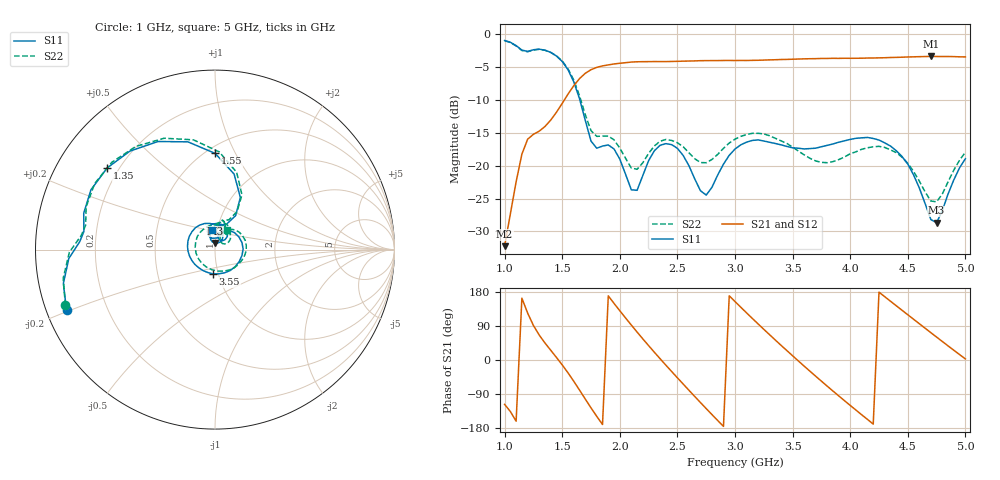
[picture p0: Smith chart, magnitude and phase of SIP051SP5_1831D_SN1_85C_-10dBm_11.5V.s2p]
# GHz  S  dB  R  50
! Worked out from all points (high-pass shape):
!   81 points, 1 GHz to 5 GHz, reference 50 ohm
!   highest |S21| = -3.41 dB at 4.7 GHz (marker M1); lowest = -32.2 dB at 1 GHz (marker M2)
!   |S21| within 3 dB of the highest: 1.673 GHz to end of sweep
!   lowest |S11| = -28.7 dB at 4.75 GHz (marker M3), VSWR 1.08, Z = 49.7 + j3.66 ohm
!   |S11| at or under -10 dB: 1.653 GHz to end of sweep
!   |S22| runs from -25.5 to -1.0 dB; largest |S21 - S12| = 0.0025
!   S11 on the Smith chart (normalised r, x): 1 GHz: 0.06, -0.20; 1.35 GHz: 0.16, +0.33; 1.55 GHz: 0.55, +0.83; 3.55 GHz: 0.94, -0.26; 5 GHz: 0.95, +0.21
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1  -0.98 -157.8  -32.24 -117.1  -32.20 -117.5  -1.01 -159.5
1.15  -2.44 176.6  -18.26 163.2  -18.23 163.2  -2.51 174.0
1.35  -2.45 142.9  -14.06 45.0  -14.07 45.0  -2.46 139.7
1.55  -5.42 89.9  -9.14 -33.8  -9.15 -33.7  -5.28 87.5
1.7  -13.10 58.7  -5.97 -103.0  -5.95 -103.0  -12.24 59.8
1.9  -16.86 81.5  -4.70 169.2  -4.68 169.3  -15.51 73.9
2.1  -23.68 81.3  -4.26 92.2  -4.26 92.2  -20.37 72.0
2.35  -16.91 96.3  -4.19 3.3  -4.18 3.3  -16.29 81.1
2.5  -17.38 63.2  -4.15 -47.0  -4.14 -47.0  -16.52 58.1
2.65  -22.00 44.7  -4.09 -96.1  -4.06 -96.0  -18.95 48.8
2.85  -21.42 77.1  -4.04 -159.7  -4.03 -159.7  -18.29 58.3
3  -17.48 52.3  -4.03 154.3  -4.01 154.2  -15.98 42.8
3.25  -16.26 -12.2  -3.96 81.0  -3.95 80.9  -15.18 -1.2
3.55  -17.36 -95.0  -3.80 -2.5  -3.79 -2.5  -17.79 -68.6
3.7  -17.35 -132.0  -3.75 -42.7  -3.74 -42.7  -19.29 -115.6
3.95  -16.24 173.3  -3.68 -107.3  -3.68 -107.3  -18.70 157.8
4.15  -15.72 131.3  -3.65 -156.8  -3.63 -156.8  -17.29 102.5
4.35  -17.03 91.4  -3.57 155.1  -3.58 155.0  -17.61 59.4
4.55  -21.41 58.9  -3.47 107.6  -3.47 107.6  -20.88 29.9
4.7  -28.20 68.9  -3.41 72.2  -3.40 72.2  -25.38 38.5
4.75  -28.69 92.6  -3.42 60.5  -3.42 60.5  -25.51 51.8
5  -18.96 97.3  -3.48 2.8  -3.48 2.7  -17.96 58.9
